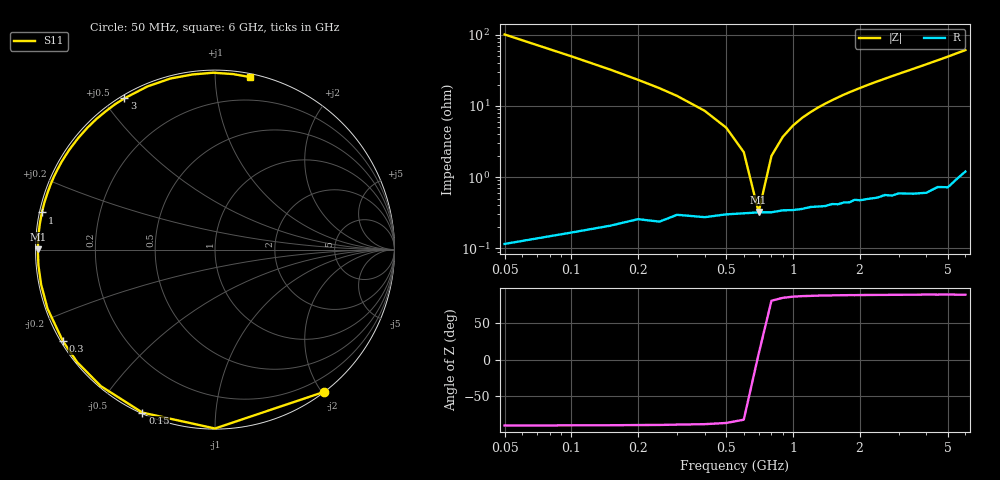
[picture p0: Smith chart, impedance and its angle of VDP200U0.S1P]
! Infineon Technologies  Discrete & RF Semiconductors
! BBY 55-03
! Si Tuning Diode in SOD323
! VR = 0.2 V
! S-Parameters:  June  1999
# GHz  S  MA  R  50
!  f  S11
! GHz  MAG  ANG
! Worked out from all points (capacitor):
!   34 points, 50 MHz to 6 GHz, reference 50 ohm
!   read as one part to ground: C = 31.2 pF near 50 MHz
!   lowest |Z| = 322 mohm at 700 MHz (marker M1)
!   series resonance near 698.1 MHz, so ESL is about 1.7 nH
!   S11 on the Smith chart (normalised r, x): 50 MHz: 0.00, -2.03; 150 MHz: 0.00, -0.65; 300 MHz: 0.01, -0.28; 1 GHz: 0.01, +0.11; 3 GHz: 0.01, +0.57; 6 GHz: 0.02, +1.22
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0.05  0.9991 -52.5
0.1  0.9967 -90.0
0.15  0.9942 -114.0
0.2  0.9916 -129.9
0.25  0.9916 -140.8
0.3  0.9891 -149.0
0.4  0.9894 -160.6
0.5  0.9882 -168.7
0.6  0.9877 -174.9
0.7  0.9873 179.9
0.8  0.9873 175.5
1  0.9865 167.9
1.1  0.9861 164.5
1.3  0.9852 158.4
1.4  0.9851 155.6
1.6  0.9846 150.3
1.8  0.984 145.3
2  0.9834 140.7
2.2  0.983 136.3
2.4  0.9829 132.2
2.8  0.9829 124.5
3  0.9823 120.9
3.5  0.9839 112.5
4  0.985 104.6
4.5  0.9838 97.3
5  0.9855 90.6
5.5  0.9831 84.2
6  0.9809 78.6
